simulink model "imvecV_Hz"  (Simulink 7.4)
settings: Solver=ode45  StartTime=0.0  StopTime=4  MaxStep=1e-3  RelTol=1e-3

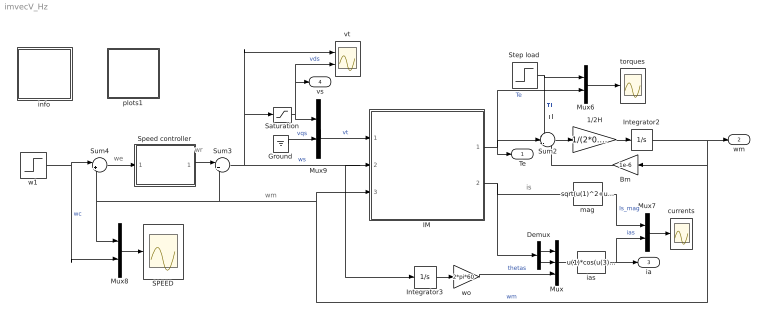
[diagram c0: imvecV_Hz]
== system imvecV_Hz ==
  note: is
  note: Tl
  note: wr
  note: we
  note: wm
  1/2H : Gain  Gain=1/(2*0.5)  ParameterDataType=sfix(16)  ParameterScaling=2^0  OutDataType=sfix(16)  OutScaling=2^0
  Bm : Gain  Gain=1e-6  ParameterDataType=sfix(16)  ParameterScaling=2^0  OutDataType=sfix(16)  OutScaling=2^0
  Demux : Demux  Outputs=2
  Ground : Ground
  IM : Subsystem  mask(Inductionmachine){Rs=0.025, Rr=0.015, Lsl=0.10, Lrl=0.10, Lm=3.0, wo=2*pi*60}
      mask prompts: Rs "Stator resistance [pu]"; Rr "Rotor resistance [pu]"; Lsl "Stator leakage inductance [pu]"; Lrl "Rotor leakage inductance [pu]"; Lm "Magnetizing inductance [pu]"; wo "Base frequency [rad/s]"
      mask help: Induction motor subsystem model using state space formulation in an arbitrary reference frame k. Parameters are expressed in per unit.
  Integrator2 : Integrator
  Integrator3 : Integrator
  Mux : Mux  Inputs=3
  Mux{6..9} (4 alike) : Mux  Inputs=2
  SPEED : Scope
  Saturation : Saturate  UpperLimit=1  LowerLimit=-1
  Speed controller : Subsystem  mask{Kp=0.6, Ki=5.6, sat=0.03}
      mask prompts: Kp "Proportional gain (Kp)"; Ki "Integral gain (Ki)"; sat "Saturation limit [pu]"
      mask help: Proportional-Integral Speed Controller
  Step load : Step  Time=2  Before=0.0  SampleTime=0
  Sum2 : Sum  Inputs=-+-  OutDataType=sfix(16)  OutScaling=2^0
  Sum3 : Sum  Inputs=|++  OutDataType=sfix(16)  OutScaling=2^0
  Sum4 : Sum  Inputs=|+-  OutDataType=sfix(16)  OutScaling=2^0
  currents : Scope
  ias : Fcn  Expr=u(1)*cos(u(3))-u(2)*sin(u(3))
  info : Subsystem
  mag : Fcn  Expr=sqrt(u(1)^2+u(2)^2)
  plots1 : Subsystem
  torques : Scope
  vt : Scope  NumInputPorts=2
  w1 : Step  Time=3  Before=1  After=0.5  SampleTime=0
  wo : Gain  Gain=2*pi*60  ParameterDataType=sfix(16)  ParameterScaling=2^0  OutDataType=sfix(16)  OutScaling=2^0
  Te : Outport
  wm : Outport  Port=2
  ia : Outport  Port=3
  vs : Outport  Port=4
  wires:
  Demux/1 -> Mux/1
  Demux/2 -> Mux/2
  mag/1 -> Mux7/1  "Is_mag"
  Sum2/1 -> 1/2H/1
  1/2H/1 -> Integrator2/1
  wo/1 -> Mux/3  "thetas"
  Bm/1 -> Sum2/3
  IM/1(Te) -> Sum2/2, Mux6/2, Te/1  "Te"
  Mux6/1 -> torques/1
  Step load/1 -> Mux6/1, Sum2/1  "Tl"
  Mux/1 -> ias/1
  Integrator3/1 -> wo/1
  Mux7/1 -> currents/1
  ias/1 -> Mux7/2, ia/1  "ias"
  IM/2(is) -> mag/1, Demux/1
  Sum4/1 -> Speed controller/1(we)
  Mux8/1 -> SPEED/1
  Ground/1 -> Mux9/2  "vqs"
  Sum3/1 -> Integrator3/1, IM/2(wk), Saturation/1, vt/1  "ws"
  Speed controller/1(wr) -> Sum3/1
  Integrator2/1 -> Bm/1, IM/3(wm), Sum4/2, Mux8/1, Sum3/2, wm/1  "wm"
  w1/1 -> Sum4/1, Mux8/2  "wc"
  Mux9/1 -> IM/1(vs)  "vt"
  Saturation/1 -> vt/2, vs/1, Mux9/1  "vds"

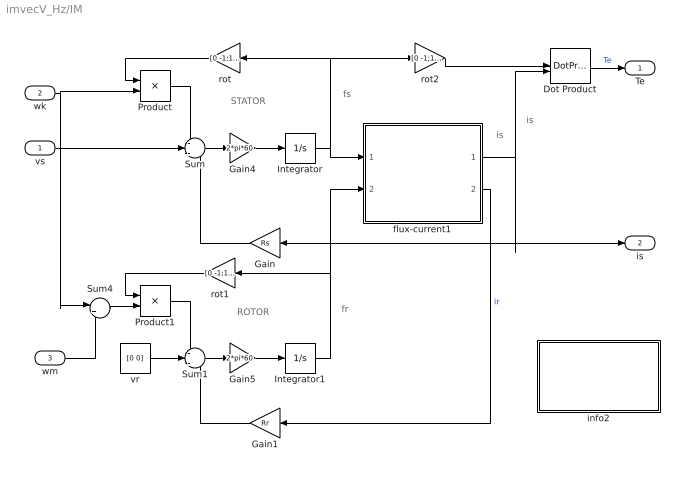
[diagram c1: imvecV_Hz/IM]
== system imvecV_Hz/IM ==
  note: ROTOR
  note: STATOR
  note: fs
  note: fr
  note: is
  note: is
  vs : Inport  OutDataType=sfix(16)  OutScaling=2^0
  wk : Inport  Port=2  OutDataType=sfix(16)  OutScaling=2^0
  wm : Inport  Port=3  OutDataType=sfix(16)  OutScaling=2^0
  Dot Product : DotProduct  OutDataType=fixdt(1, 16)  OutScaling=2^-10
  Gain : Gain  Gain=Rs  ParameterDataType=sfix(16)  ParameterScaling=2^0  OutDataType=sfix(16)  OutScaling=2^0
  Gain1 : Gain  Gain=Rr  ParameterDataType=sfix(16)  ParameterScaling=2^0  OutDataType=sfix(16)  OutScaling=2^0
  Gain4 : Gain  Gain=2*pi*60  ParameterDataType=sfix(16)  ParameterScaling=2^0  OutDataType=sfix(16)  OutScaling=2^0
  Gain5 : Gain  Gain=2*pi*60  ParameterDataType=sfix(16)  ParameterScaling=2^0  OutDataType=sfix(16)  OutScaling=2^0
  Integrator : Integrator  InitialCondition=[0 0]
  Integrator1 : Integrator  InitialCondition=[0 0]
  Product : Product  OutDataType=sfix(16)  OutScaling=2^0
  Product1 : Product  OutDataType=sfix(16)  OutScaling=2^0
  Sum : Sum  Inputs=-+-  OutDataType=sfix(16)  OutScaling=2^0
  Sum1 : Sum  Inputs=-+-  OutDataType=sfix(16)  OutScaling=2^0
  Sum4 : Sum  Inputs=|+-  OutDataType=sfix(16)  OutScaling=2^0
  flux-current1 : Subsystem
  info2 : Subsystem
  rot : Gain  Gain=[0 -1;1 0]  Multiplication=Matrix(K*u)  ParameterDataType=sfix(16)  ParameterScaling=2^0  OutDataType=sfix(16)  OutScaling=2^0
  rot1 : Gain  Gain=[0 -1;1 0]  Multiplication=Matrix(K*u)  ParameterDataType=sfix(16)  ParameterScaling=2^0  OutDataType=sfix(16)  OutScaling=2^0
  rot2 : Gain  Gain=[0 -1;1 0]  Multiplication=Matrix(K*u)  ParameterDataType=sfix(16)  ParameterScaling=2^0  OutDataType=sfix(16)  OutScaling=2^0
  vr : Constant  Value=[0 0]  OutDataType=sfix(16)  OutScaling=2^0
  Te : Outport
  is : Outport  Port=2
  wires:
  Gain/1 -> Sum/3
  vr/1 -> Sum1/2
  Gain1/1 -> Sum1/3
  flux-current1/2(ir) -> Gain1/1  "ir"
  Integrator/1 -> flux-current1/1(fs), rot/1, rot2/1
  Integrator1/1 -> flux-current1/2(fr), rot1/1
  Product1/1 -> Sum1/1
  rot1/1 -> Product1/1
  Product/1 -> Sum/1
  rot/1 -> Product/1
  rot2/1 -> Dot Product/1
  Sum4/1 -> Product1/2
  Sum/1 -> Gain4/1
  Gain4/1 -> Integrator/1
  Sum1/1 -> Gain5/1
  Gain5/1 -> Integrator1/1
  flux-current1/1(is) -> Gain/1, is/1, Dot Product/2
  Dot Product/1 -> Te/1  "Te"
  vs/1 -> Sum/2
  wk/1 -> Product/2, Sum4/1
  wm/1 -> Sum4/2

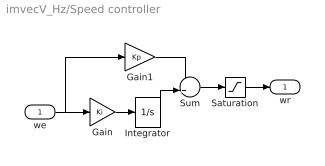
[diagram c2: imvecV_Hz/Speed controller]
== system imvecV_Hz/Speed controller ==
  we : Inport  OutDataType=sfix(16)  OutScaling=2^0
  Gain : Gain  Gain=Ki  ParameterDataType=sfix(16)  ParameterScaling=2^0  OutDataType=sfix(16)  OutScaling=2^0
  Gain1 : Gain  Gain=Kp  ParameterDataType=sfix(16)  ParameterScaling=2^0  OutDataType=sfix(16)  OutScaling=2^0
  Integrator : Integrator  LimitOutput=on  UpperSaturationLimit=sat  LowerSaturationLimit=-sat
  Saturation : Saturate  UpperLimit=sat  LowerLimit=-sat
  Sum : Sum  OutDataType=sfix(16)  OutScaling=2^0
  wr : Outport  InitialOutput=0
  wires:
  Saturation/1 -> wr/1
  Sum/1 -> Saturation/1
  Integrator/1 -> Sum/2
  we/1 -> Gain1/1, Gain/1
  Gain/1 -> Integrator/1
  Gain1/1 -> Sum/1

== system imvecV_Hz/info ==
  note: Volts/Hz closed-loop speed control of an induction motor {dq model} [pu]
  note: To modify the machine parameters, double click the induction motor block. To adjust the speed controller, double click the PI block. To run an identical operation of the induction motor modeled in abc phase variables, access the file named .

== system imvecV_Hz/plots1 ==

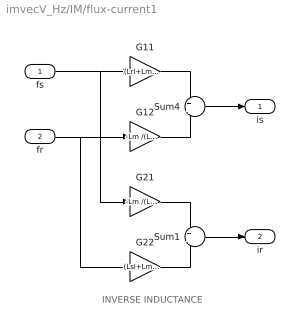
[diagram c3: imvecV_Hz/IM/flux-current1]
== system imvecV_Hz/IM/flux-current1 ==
  note: INVERSE INDUCTANCE
  fs : Inport  OutDataType=sfix(16)  OutScaling=2^0
  fr : Inport  Port=2  OutDataType=sfix(16)  OutScaling=2^0
  G11 : Gain  Gain=(Lrl+Lm) /(Lsl*Lrl+Lsl*Lm+Lrl*Lm)  ParameterDataType=sfix(16)  ParameterScaling=2^0  OutDataType=sfix(16)  OutScaling=2^0
  G12 : Gain  Gain=-Lm /(Lsl*Lrl+Lsl*Lm+Lrl*Lm)  ParameterDataType=sfix(16)  ParameterScaling=2^0  OutDataType=sfix(16)  OutScaling=2^0
  G21 : Gain  Gain=-Lm /(Lsl*Lrl+Lsl*Lm+Lrl*Lm)  ParameterDataType=sfix(16)  ParameterScaling=2^0  OutDataType=sfix(16)  OutScaling=2^0
  G22 : Gain  Gain=(Lsl+Lm )/(Lsl*Lrl+Lsl*Lm+Lrl*Lm)  ParameterDataType=sfix(16)  ParameterScaling=2^0  OutDataType=sfix(16)  OutScaling=2^0
  Sum1 : Sum  OutDataType=sfix(16)  OutScaling=2^0
  Sum4 : Sum  OutDataType=sfix(16)  OutScaling=2^0
  is : Outport
  ir : Outport  Port=2
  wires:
  fs/1 -> G11/1, G21/1
  G11/1 -> Sum4/1
  fr/1 -> G12/1, G22/1
  G12/1 -> Sum4/2
  Sum4/1 -> is/1
  G21/1 -> Sum1/1
  G22/1 -> Sum1/2
  Sum1/1 -> ir/1

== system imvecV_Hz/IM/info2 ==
  note: Synchronous machine transients under shortcircuit
  note: This demonstration illustrates the dynamics of a synchronous generator, initially at no load, following a three-phase short circuit at the terminals.
